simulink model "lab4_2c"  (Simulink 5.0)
settings: Solver=FixedStepDiscrete  StartTime=0.0  StopTime=2*1e-3  FixedStep=T  RelTol=1e-3
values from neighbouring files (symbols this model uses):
  T = 1/Fsamp    (= 0.0001)    [lab4_4.m]

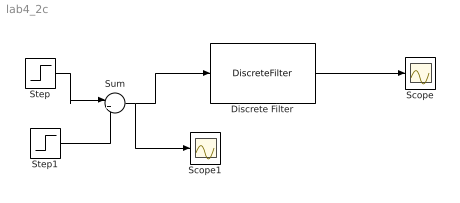
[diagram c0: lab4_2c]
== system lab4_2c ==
  Discrete Filter : DiscreteFilter  Numerator="[2  1]"  Denominator="[1  -1.8*cos(pi/16)  0.81]"  SampleTime=T
  Scope : Scope
  Scope1 : Scope
  Step : Step  Time=0  Before=1  SampleTime=T
  Step1 : Step  Time=0  Before=1  SampleTime=T
  Sum : Sum  Inputs=|+-
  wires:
  Discrete Filter/1 -> Scope/1
  Step/1 -> Sum/1
  Sum/1 -> Discrete Filter/1, Scope1/1
  Step1/1 -> Sum/2
